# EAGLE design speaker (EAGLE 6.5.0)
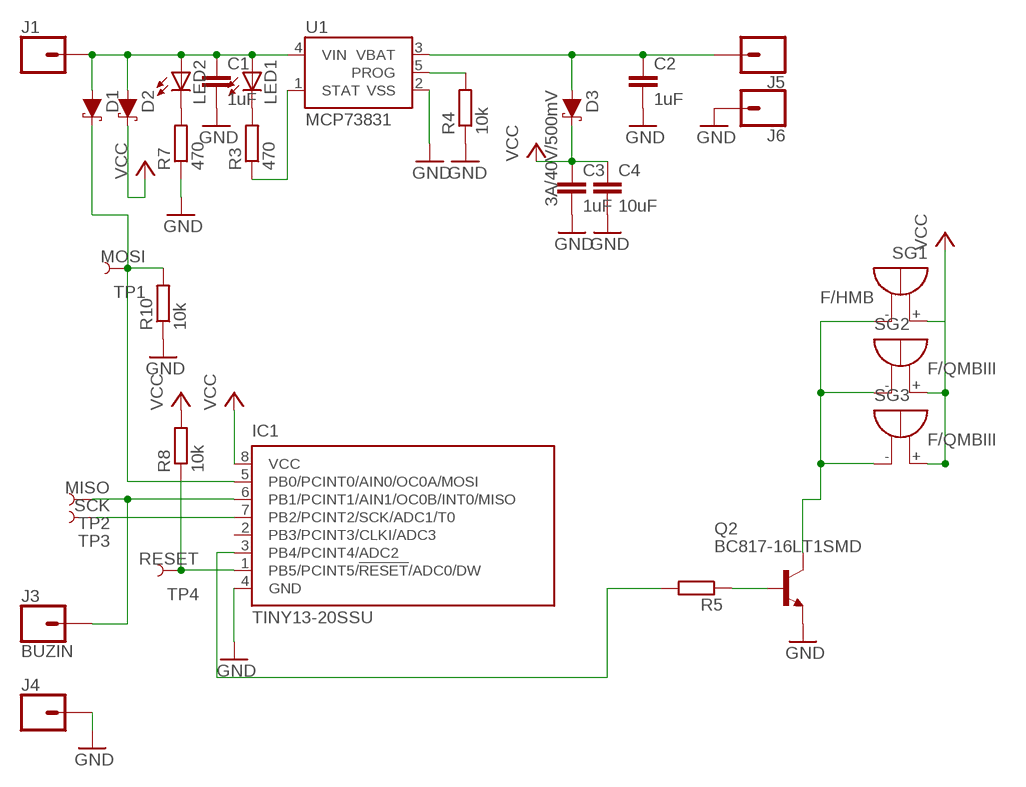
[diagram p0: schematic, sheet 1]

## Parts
C1  1uF  C-EUC1206  [C1206]
C2  1uF  C-EUC1206  [C1206]
C3  1uF  C-EUC1206  [C1206]
C4  10uF  C-EUC1206  [C1206]
D1  DIODE-SCHOTTKY-B340A  [SMA-DIODE]
D2  DIODE-SCHOTTKY-B340A  [SMA-DIODE]
D3  3A/40V/500mV  DIODE-SCHOTTKY-B340A  [SMA-DIODE]
IC1  TINY13-20SSU  [8S1]
J1  CONN_01OFFSET  [1X01_OFFSET]
J3  BUZIN  CONN_01OFFSET  [1X01_OFFSET]
J4  CONN_01OFFSET  [1X01_OFFSET]
J5  CONN_01OFFSET  [1X01_OFFSET]
J6  CONN_01OFFSET  [1X01_OFFSET]
LED1  LEDCHIP-LED0805  [CHIP-LED0805]
LED2  LEDCHIP-LED0805  [CHIP-LED0805]
Q2  BC817-16LT1SMD  [SOT23-BEC]
R3  470  R-EU_M0805  [M0805]
R4  10k  R-EU_M0805  [M0805]
R5  R-EU_M0805  [M0805]
R7  470  R-EU_M0805  [M0805]
R8  10k  R-EU_M0805  [M0805]
R10  10k  R-EU_M0805  [M0805]
SG1  F/HMB  [F/HMB]
SG2  F/QMBIII  [F/QMBIII]
SG3  F/QMBIII  [F/QMBIII]
TP1  MOSI  TEST-POINT3X5  [PAD.03X.05]
TP2  MISO  TEST-POINT3X5  [PAD.03X.05]
TP3  SCK  TEST-POINT3X5  [PAD.03X.05]
TP4  RESET  TEST-POINT3X5  [PAD.03X.05]
U1  MCP73831  [SOT23-5]

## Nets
BUZER: Q2.C SG1.- SG2.-(+) SG3.-(+)
GND: C1.2 C2.2 C3.2 C4.2 IC1.4(GND) J4.1 J6.1 Q2.E R4.1 R7.1 R10.1 U1.2(VSS)
N$1: LED2.C R7.2
N$3: C1.1 D1.A D2.A J1.1 LED1.A LED2.A U1.4(VIN)
N$4: LED1.C R3.2
N$6: R3.1 U1.1(STAT)
N$7: R4.2 U1.5(PROG)
N$8: C2.1 D3.A J5.1 U1.3(VBAT)
N$9: IC1.6(PB1/PCINT1/AIN1/OC0B/INT0/MISO) J3.1 TP2.P$1
N$10: IC1.1(PB5/PCINT5/!RESET!/ADC0/DW) R8.1 TP4.P$1
N$12: D1.C IC1.5(PB0/PCINT0/AIN0/OC0A/MOSI) R10.2 TP1.P$1
N$13: IC1.7(PB2/PCINT2/SCK/ADC1/T0) TP3.P$1
N$18: Q2.B R5.1
N$20: IC1.3(PB4/PCINT4/ADC2) R5.2
VCC: C3.1 C4.1 D2.C D3.C IC1.8(VCC) R8.2 SG1.+ SG2.+(-) SG3.+(-)
Unconnected: IC1.2(PB3/PCINT3/CLKI/ADC3)

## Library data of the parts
C1-C4 = rcl:C-EU: CAPACITOR, European symbol
D1 D2 = SparkFun-DiscreteSemi:DIODE-SCHOTTKY: Schottky diode; PROD_ID: DIO-09886; VALUE: 3A/40V/500mV
D3 = SparkFun-DiscreteSemi:DIODE-SCHOTTKY: Schottky diode; PROD_ID: DIO-09886
IC1 = atmel:TINY13: 8-bit AVR Microcontroller with 1K Bytes In-System Programmable Flash Source: http://www.atmel.com/dyn/resources/prod_documents/2535S.pdf; MPN: ATTINY13-20SSU; OC_FARNELL: 1455133; OC_NEWARK: 58M3771
J1 J3-J6 = SparkFun-Connectors:CONN_01: Single connection point. Often used as Generic Header-pin footprint for 0.1 inch spaced/style header connections
LED1 LED2 = led:LED: LED
Q2 = transistor-npn:BC817*: NPN Transistor
R3-R5 R7 R8 R10 = rcl:R-EU_: RESISTOR, European symbol
SG1 = buzzer:F/HMB: BUZZER; OC_FARNELL: unknown; OC_NEWARK: unknown
SG2 SG3 = buzzer:F/QMBIII: BUZZER; OC_FARNELL: unknown; OC_NEWARK: unknown
TP1-TP4 = SparkFun-Connectors:TEST-POINT: SparkFun Test Points
U1 = SparkFun-IC-Power:MCP73831: MCP73831T Li-Ion, Li-Pol Controller Miniature single cell, fully integrated Li-Ion, Li-polymer charge management controller Datasheet SparkFun Products: SparkFun ESP32 Thing SparkFun 9DoF Razor IMU M0; PROD_ID: IC-09995

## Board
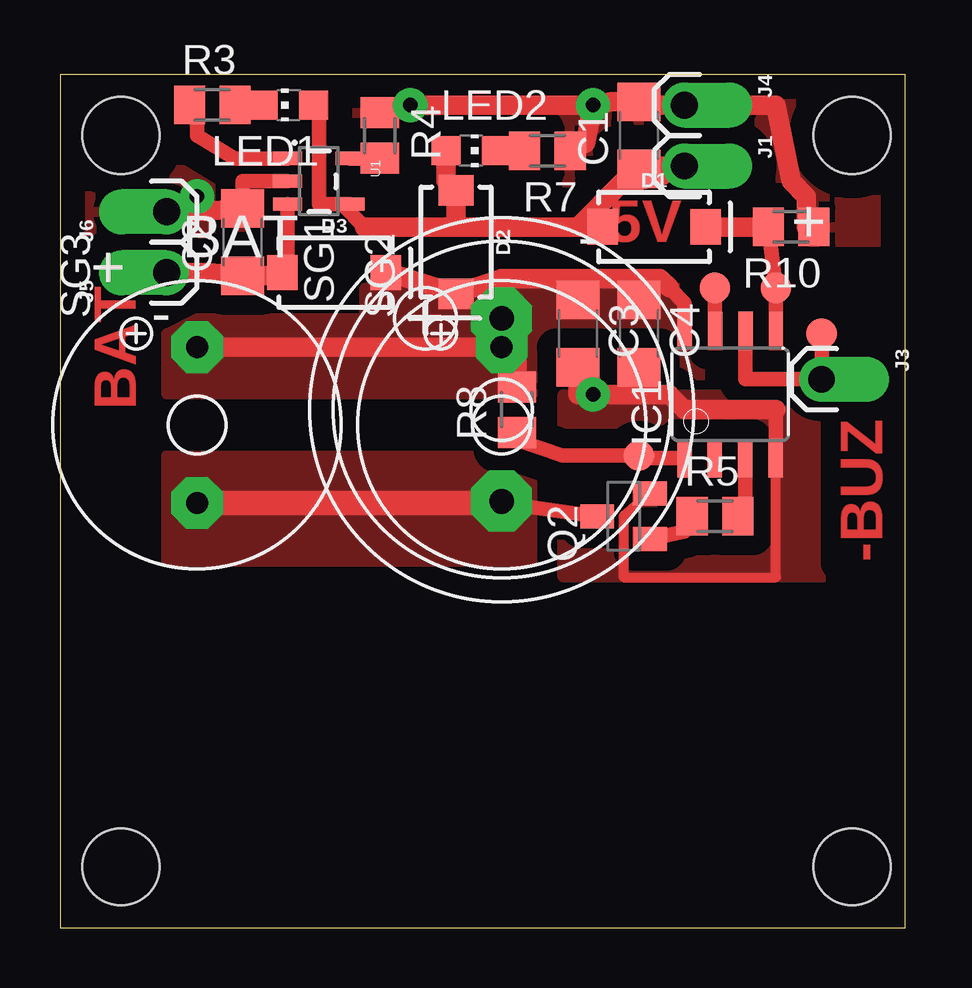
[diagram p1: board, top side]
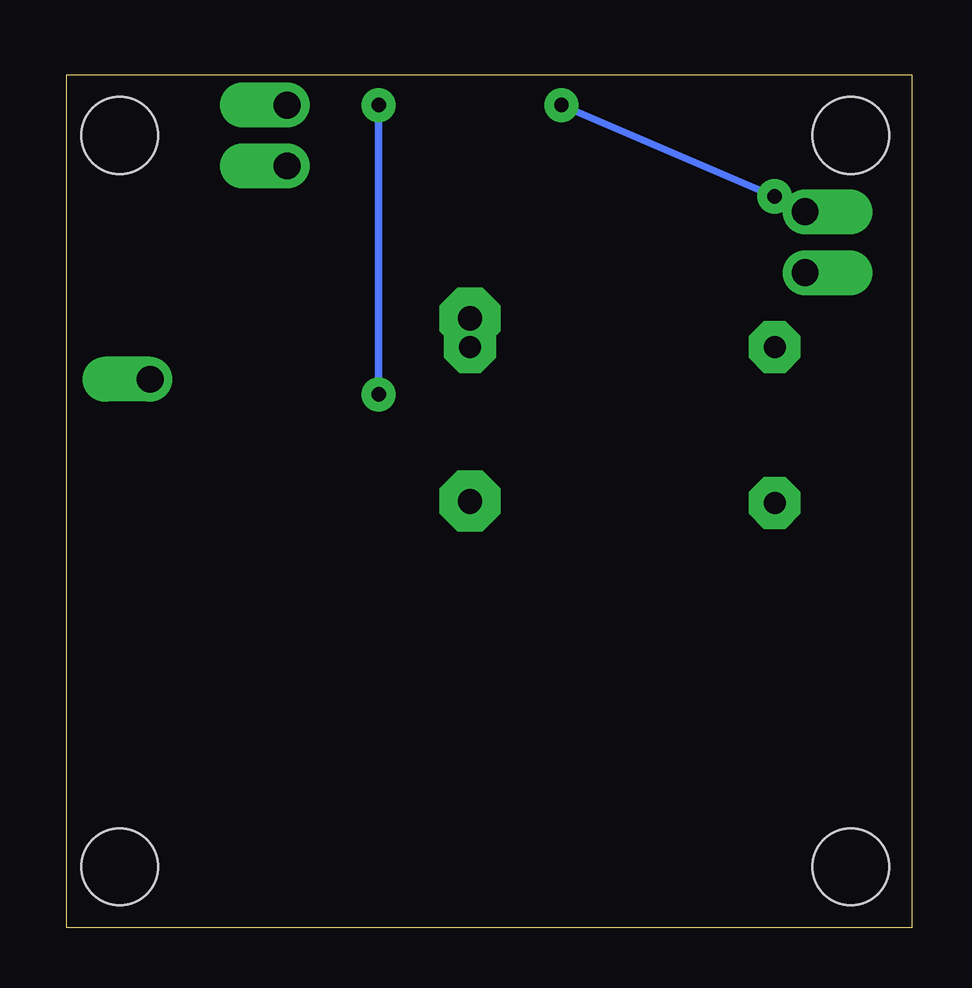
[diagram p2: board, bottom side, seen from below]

Size 35.23 x 35.55 mm. Coordinates in mm from the lower left corner, seen from the top.
Outline: 0,0 35.23,0 35.23,35.55 0,35.55 0,0
Copper layers (1*16): Top 0.035mm / dielectric 1.5mm / Bottom 0.035mm
Design rules "default": minimum track width 10mil, minimum drill 24mil, track to track 8mil, track to pad 8mil, pad to pad 8mil, via to via 8mil, smd to smd 8mil, copper to edge 40mil, drill to drill 8mil, minimum pad ring 10mil, minimum via ring 8mil, stop-mask expansion 4mil, vias tented up to drill 0mil, thermal gap 10mil
Holes 3.2 mm at 2.54,2.54 33.02,2.54 33.02,33.02 2.54,33.02

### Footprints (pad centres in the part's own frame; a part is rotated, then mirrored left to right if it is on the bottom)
C1206 = smd 1.6 x 1.8: 1 -1.4,0; 2 1.4,0
SMA-DIODE = smd 1.27 x 1.47: A -2.15,0; C 2.15,0
8S1 = smd 0.6 x 1.6: 1 -1.905,-2.654; 2 -0.645,-2.654; 3 0.625,-2.654; 4 1.895,-2.654; 5 1.905,2.654; 6 0.635,2.654; 7 -0.635,2.654; 8 -1.905,2.654
1X01_OFFSET = drill 1.118 pad 1.88 offset: 1 0,0
CHIP-LED0805 = smd 1.2 x 1.2: A 0,-1.05; C 0,1.05
SOT23-BEC = smd 1 x 1.4: B -0.95,-1.1; C 0,1.1; E 0.95,-1.1
M0805 = smd 1.3 x 1.6: 1 -0.95,0; 2 0.95,0
F/HMB = drill 1.016 pad 2.54 octagon: + 3.81,0; - -3.81,0
F/QMBIII = drill 0.914 pad 2.159 octagon: + 3.251,0; - -3.251,0
PAD.03X.05 = smd 1.27 x 1.27: P$1 0,0
SOT23-5 = smd 0.55 x 1.2: 1 -0.95,-1.3; 2 0,-1.3; 3 0.95,-1.3; 4 0.95,1.3; 5 -0.95,1.3

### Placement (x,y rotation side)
C1  24.13,33.02 90 top
C2  7.62,28.57 90 top
C3  21.59,24.77 270 top
C4  24.13,24.77 270 top
D1  24.77,29.21 0 top
D2  16.51,28.57 270 top
D3  11.43,27.3 0 top
IC1  27.94,22.23 0 top
J1  26.04,31.75 270 top
J3  31.75,22.86 270 top
J4  26.04,34.29 270 top
J5  4.45,27.3 90 top
J6  4.45,29.84 90 top
LED1  9.53,34.29 90 top
LED2  17.14,32.38 270 top
Q2  23.5,17.14 90 top
R3  6.35,34.29 0 top
R4  13.34,33.02 270 top
R5  27.3,17.14 0 top
R7  20.32,32.38 180 top
R8  19.05,21.59 90 top
R10  30.48,29.21 180 top
SG1  18.41,21.59 90 top
SG2  18.41,20.95 90 top
SG3  5.71,20.95 90 top
TP1  29.84,26.67 0 top
TP2  31.75,24.77 0 top
TP3  27.3,26.67 0 top
TP4  24.13,19.68 0 top
U1  10.79,31.11 270 top

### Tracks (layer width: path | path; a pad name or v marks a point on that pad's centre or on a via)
BUZER
  Top 0.61: Q2.C SG2.-
  Top 1.016: SG2.- SG3.-
  pour Top (isolate 1.016, no thermals): 4.45,19.68 19.68,19.68 19.68,15.24 4.45,15.24
GND  (via drill 0.6 pad 1.42)
  Top 0.406: Q2.E 23.5,17.14 23.5,14.61 29.84,14.61 29.84,19.05
  Top 0.61: U1.2 7.62,31.11 C2.2 | 29.84,21.59 IC1.4 29.84,19.05 | R10.1 31.11,29.21
  Top 0.813: 31.11,29.21 31.11,30.48 30.48,31.11 29.84,34.29 J4.1 24.89,34.29 C1.2 22.99,34.42 | 24.13,22.23 C4.2 | 29.84,21.59 26.04,21.59 25.4,22.23 24.13,22.23 | C3.2 21.59,22.23 v22.23,22.23 24.13,22.23 | 22.99,34.42 v22.23,34.29 21.91,32.7 R7.1 | 22.99,34.42 21.85,34.29 v14.61,34.29 R4.1 | v5.71,30.48 5.71,29.84 | J6.1 5.71,29.84 | 5.71,29.84 C2.2
  Bottom 0.305: v22.23,34.29 v22.23,22.23 | v14.61,34.29 v5.71,30.48
  pour Top (isolate 0.813, no thermals): 20.95,22.23 34.29,22.23 34.29,14.61 20.95,14.61
  pour Top (isolate 1.016): 0.64,34.92 34.92,34.92 34.92,28.57 0.64,28.57
N$1
  Top 0.813: LED2.C R7.2
N$3
  Top 0.61: LED1.A 10.79,34.29 10.79,30.16 U1.4 11.75,30.16 12.7,29.21
  Top 0.813: 16.51,29.21 12.7,29.21 | J1.1 24.89,31.75 C1.1 25.14,31.36 24.13,31.11 23.5,31.11 21.59,29.21 D1.A 16.51,29.21 | 16.51,29.21 D2.A 16.09,31.14 LED2.A
N$4
  Top 0.61: R3.2 LED1.C
N$6
  Top 0.61: U1.1 7.3,32.06 5.71,33.02 5.71,34.29 R3.1
N$7
  Top 0.61: U1.5 13.02,32.06 R4.2
N$8
  Top 0.61: U1.3 9.49,27.2 8.26,27.18
  Top 0.813: J5.1 6.22,27.3 C2.1 8.26,27.18 9.15,27.18 D3.A
N$9
  Top 0.61: IC1.6 28.57,22.86 J3.1 TP2.P$1
N$10
  Top 0.61: IC1.1 24.13,19.57 TP4.P$1 20.95,19.68 19.05,20.32 R8.1
N$12
  Top 0.61: IC1.5 TP1.P$1 R10.2
  Top 0.813: R10.2 D1.C
N$13
  Top 0.61: TP3.P$1 IC1.7
N$18
  Top 0.61: Q2.B 26.04,16.51 R5.1
N$20
  Top 0.61: IC1.3 28.57,17.78 R5.2
VCC
  Top 0.61: IC1.8 26.04,26.04 25.4,26.67 | C4.1 24.13,27.06 | C3.1 21.59,27.06
  Top 0.813: SG3.+ SG2.+ | D3.C 13.72,27.3 D2.C 18.41,27.06 | R8.2 19.05,23.57 SG2.+ | SG2.+ SG1.+ 18.41,27.06 | 18.41,27.06 21.59,27.06 24.13,27.06 25.01,27.06 25.4,26.67
  pour Top (isolate 0.813, no thermals): 5.71,25.4 12.7,25.4 12.7,26.67 26.67,26.67 26.67,22.23 4.45,22.23 4.45,24.77

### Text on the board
Top: 5V | BAT | -BUZ
tNames: + | BAT | - | + | -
